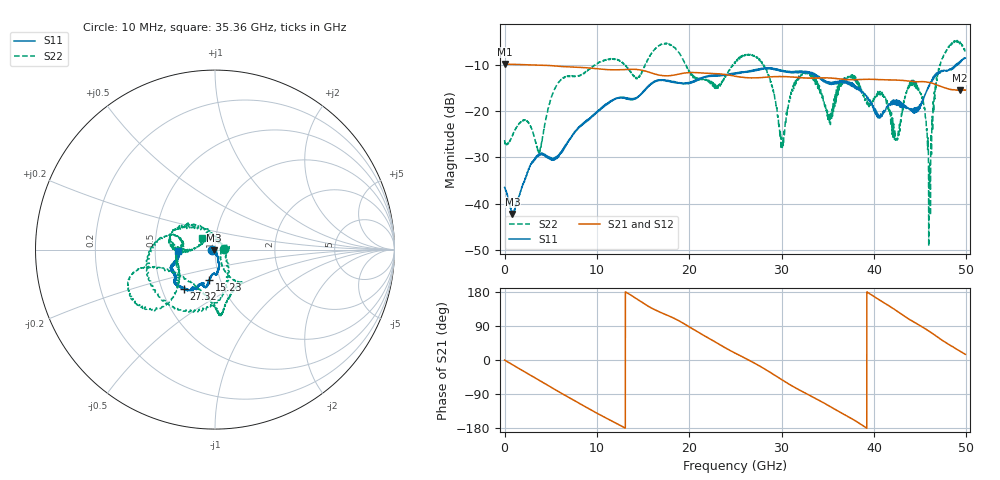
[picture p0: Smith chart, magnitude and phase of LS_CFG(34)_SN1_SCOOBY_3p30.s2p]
!Keysight Technologies,N5245B,MY58422026,A.13.80.08
!Date: Thursday, March 19, 2020 23:37:27
!Correction: S11(Full 2 Port(1,2))
!S21(Full 2 Port(1,2))
!S12(Full 2 Port(1,2))
!S22(Full 2 Port(1,2))
!S2P File: Measurements: S11, S21, S12, S22:
# Hz S DB R 50.0
!freq dBS11 angS11 dBS21 angS21 dBS12 angS12 dBS22 angS22
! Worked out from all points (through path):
!   4991 points, 10 MHz to 49.91 GHz, reference 50 ohm
!   highest |S21| = -9.83 dB at 10 MHz (marker M1); lowest = -15.5 dB at 49.34 GHz (marker M2)
!   group delay of S21, straight-line fit = 38.6 ps
!   lowest |S11| = -42.3 dB at 850 MHz (marker M3), VSWR 1.02, Z = 49.4 - j0.465 ohm
!   |S11| at or under -10 dB: start of sweep to 48.89 GHz; 48.9376 GHz to 48.99048 GHz (52.88 MHz wide, 0.108 % of centre)
!   |S22| runs from -49.2 to -4.7 dB; largest |S21 - S12| = 0.0029
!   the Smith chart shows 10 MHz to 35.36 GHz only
!   S11 on the Smith chart (normalised r, x): 10 MHz: 0.97, -0.01; 15.23 GHz: 0.89, -0.31; 27.32 GHz: 0.65, -0.30; 35.36 GHz: 0.66, -0.02
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1e7  -36.52 -169.0  -9.83 -0.3  -9.82 -0.3  -26.27 0.9
8.5e8  -42.28 -142.2  -9.89 -12.3  -9.88 -12.3  -25.25 -11.5
3.77e9  -29.48 -71.6  -10.04 -53.8  -10.04 -53.7  -28.49 -20.5
5.63e9  -29.93 -74.0  -10.27 -80.5  -10.26 -80.5  -14.46 -59.3
8.33e9  -23.19 -74.9  -10.55 -117.6  -10.54 -117.6  -12.14 -64.1
1.523e10  -15.32 -101.0  -11.35 146.7  -11.33 146.7  -9.95 -160.9
1.665e10  -13.40 -104.0  -12.16 128.2  -12.16 128.2  -5.95 -160.8
2.289e10  -12.44 -116.0  -11.89 46.6  -11.89 46.8  -15.10 174.4
2.496e10  -11.93 -120.6  -12.44 18.3  -12.42 18.5  -9.59 175.7
2.732e10  -11.09 -128.8  -12.80 -11.7  -12.79 -11.5  -8.53 -115.8
3.003e10  -11.26 -145.0  -12.57 -52.1  -12.56 -51.9  -27.04 23.5
3.139e10  -11.46 -149.8  -12.67 -71.9  -12.68 -71.7  -13.83 137.2
3.328e10  -11.81 -160.8  -12.86 -96.5  -12.86 -96.2  -12.31 176.5
3.536e10  -13.81 -176.7  -12.88 -124.3  -12.82 -124.0  -20.41 138.7
3.735e10  -14.14 167.2  -13.19 -151.6  -13.10 -151.7  -12.55 141.0
4.16e10  -18.51 99.9  -13.26 143.4  -13.28 143.3  -19.65 31.5
4.245e10  -17.84 99.7  -13.30 130.1  -13.32 129.8  -25.64 -14.8
4.457e10  -19.53 44.6  -13.65 96.9  -13.68 96.9  -14.09 -12.4
4.602e10  -14.47 5.7  -13.80 75.2  -13.82 75.3  -34.79 82.7
4.711e10  -11.40 8.1  -14.56 56.9  -14.57 57.0  -10.28 -98.9
4.934e10  -9.45 -19.5  -15.52 23.0  -15.54 23.2  -5.04 -33.0
4.991e10  -8.52 -17.0  -15.45 15.0  -15.48 14.9  -7.18 -19.3
